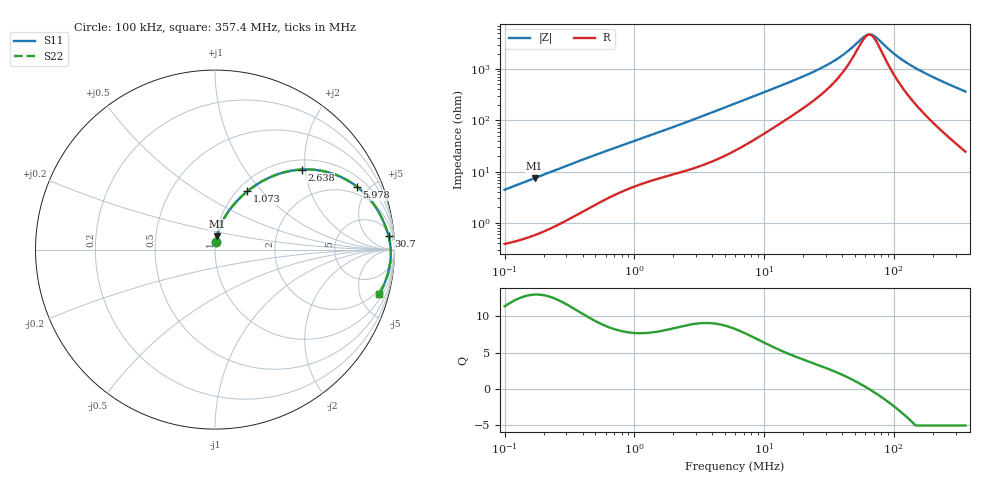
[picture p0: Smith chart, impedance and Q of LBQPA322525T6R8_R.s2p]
! LBQPA322525T6R8_R  S-PARAMETER MODEL  ( General Type )
! Model Generated by TAIYO YUDEN Corporation (http://www.ty-top.com)
! Version 1.0
! TAIYO YUDEN Control No. 191025NI43SB-FBB
! Copyright(c) 2019 TAIYO YUDEN CO.,LTD. All Rights Reserved.
! Product Description (link to TY-COMPAS)
! https://ds.yuden.co.jp/TYCOMPAS/or/detail?pn=LBQPA322525T6R8MR&u=M
! Products Name : Inductors
! Characteristics :
!  Inductance : 6.8 uH , SRF(min) : 50 MHz , DC Resistance(max) : 0.156 Ohm
!  Rated Current : Saturation :950 mA , Temp Rise : 760 mA (20 degC)
!  Case Size : 3.2 x 2.5 / 0.126 x 0.098 [mm/inch] , Thickness : 2.5 / 0.098 [mm/inch]
!  (Conditions: Temperature = 25 degC , DC Bias Current/Voltage = 0A / 0V)
! External Node Assignments :
!  1  o---GGG---o  2
! GND o---------o GND
! Frequency Range : 0.1MHz  -  357.398349MHz  [ 402 STEP ]
# MHz S RI R 50
! Freq[MHz].  S11 Real  S11 Imag  S21 Real  S21 Imag  S12 Real  S12 Imag  S22 Real  S22 Imag
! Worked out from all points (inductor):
!   401 points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, 100 kHz to 357.4 MHz, reference 50 ohm
!   read as one part in series: L = 7 uH near 104.2 kHz
!   highest Q = 12.9 at 170.2 kHz (marker M1), where L = 6.97 uH
!   self-resonance near 64.6 MHz
!   S11 on the Smith chart (normalised r, x): 100 kHz: 1.01, +0.09; 1.073 MHz: 1.11, +0.84; 2.638 MHz: 1.22, +1.91; 5.978 MHz: 1.51, +4.22; 30.7 MHz: 9, +23; 357.4 MHz: 1.49, -7.28
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0.1  0.00581 0.0438  0.9942 -0.0438  0.9942 -0.0438  0.00581 0.0438
0.170198  0.0112 0.0733  0.9888 -0.0733  0.9888 -0.0733  0.0112 0.0733
0.393689  0.0421 0.1582  0.9579 -0.1582  0.9579 -0.1582  0.0421 0.1582
0.670051  0.0957 0.2401  0.9043 -0.2401  0.9043 -0.2401  0.0957 0.2401
1.072542  0.1803 0.3246  0.8197 -0.3246  0.8197 -0.3246  0.1803 0.3246
1.549909  0.2799 0.3901  0.7201 -0.3901  0.7201 -0.3901  0.2799 0.3901
2.637916  0.4821 0.4461  0.5179 -0.4461  0.5179 -0.4461  0.4821 0.4461
3.812  0.6375 0.4286  0.3625 -0.4286  0.3625 -0.4286  0.6375 0.4286
5.97828  0.7914 0.3501  0.2086 -0.3501  0.2086 -0.3501  0.7914 0.3501
6.101817  0.7969 0.3458  0.2031 -0.3458  0.2031 -0.3458  0.7969 0.3458
10.81882  0.9033 0.2245  0.0967 -0.2245  0.0967 -0.2245  0.9033 0.2245
23.53582  0.9583 0.1042  0.0417 -0.1042  0.0417 -0.1042  0.9583 0.1042
30.70484  0.9673 0.0738  0.0327 -0.0738  0.0327 -0.0738  0.9673 0.0738
40.88529  0.9739 0.0442  0.0261 -0.0442  0.0261 -0.0442  0.9739 0.0442
57.88634  0.9785 0.0105  0.0215 -0.0105  0.0215 -0.0105  0.9785 0.0105
62.8214  0.979 0.00268  0.021 -0.00268  0.021 -0.00268  0.979 0.00268
71.02397  0.9796 -0.00917  0.0204 0.00917  0.0204 0.00917  0.9796 -0.00917
92.65788  0.9793 -0.0358  0.0207 0.0358  0.0207 0.0358  0.9793 -0.0358
118.4342  0.9771 -0.0628  0.0229 0.0628  0.0229 0.0628  0.9771 -0.0628
157.702  0.9715 -0.0987  0.0285 0.0987  0.0285 0.0987  0.9715 -0.0987
237.4078  0.9541 -0.1628  0.0459 0.1628  0.0459 0.1628  0.9541 -0.1628
357.3983  0.9159 -0.246  0.0841 0.246  0.0841 0.246  0.9159 -0.246
